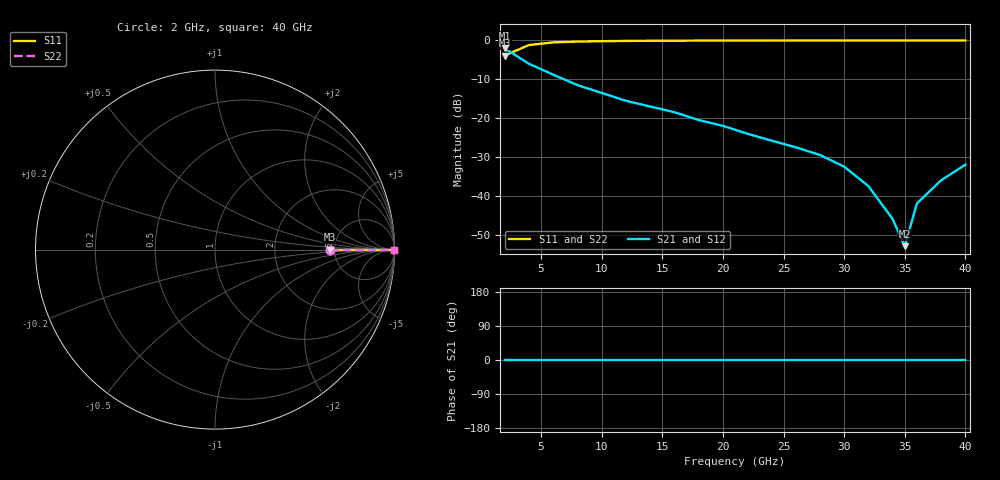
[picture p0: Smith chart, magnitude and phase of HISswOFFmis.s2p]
# GHZ S MA R 50
!Output file by Shape3_28
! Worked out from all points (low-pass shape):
!   21 points, 2 GHz to 40 GHz, reference 50 ohm
!   highest |S21| = -2.04 dB at 2 GHz (marker M1); lowest = -53.0 dB at 35 GHz (marker M2)
!   |S21| within 3 dB of the highest: start of sweep to 3.513 GHz
!   lowest |S11| = -3.9 dB at 2 GHz (marker M3), VSWR 4.52, Z = 226 + j0 ohm
!   |S11| at or under -10 dB: nowhere
!   |S22| runs from -3.9 to 0.0 dB; largest |S21 - S12| = 0
2  0.638 0.0  0.791 0.0  0.791 0.0  0.638 0.0
4  0.871 0.0  0.501 0.0  0.501 0.0  0.871 0.0
6  0.944 0.0  0.363 0.0  0.363 0.0  0.944 0.0
8  0.966 0.0  0.266 0.0  0.266 0.0  0.966 0.0
10  0.977 0.0  0.211 0.0  0.211 0.0  0.977 0.0
12  0.985 0.0  0.167 0.0  0.167 0.0  0.985 0.0
14  0.99 0.0  0.141 0.0  0.141 0.0  0.99 0.0
16  0.992 0.0  0.119 0.0  0.119 0.0  0.992 0.0
18  0.994 0.0  0.0944 0.0  0.0944 0.0  0.994 0.0
20  0.996 0.0  0.0794 0.0  0.0794 0.0  0.996 0.0
22  0.997 0.0  0.063 0.0  0.063 0.0  0.997 0.0
24  0.9975 0.0  0.0513 0.0  0.0513 0.0  0.9975 0.0
26  0.998 0.0  0.0421 0.0  0.0421 0.0  0.998 0.0
28  0.9985 0.0  0.0335 0.0  0.0335 0.0  0.9985 0.0
30  0.9986 0.0  0.0237 0.0  0.0237 0.0  0.9986 0.0
32  0.9988 0.0  0.0133 0.0  0.0133 0.0  0.9988 0.0
34  0.9989 0.0  0.005012 0.0  0.005012 0.0  0.9989 0.0
35  0.999 0.0  0.002239 0.0  0.002239 0.0  0.999 0.0
36  0.9989 0.0  0.007943 0.0  0.007943 0.0  0.9989 0.0
38  0.9988 0.0  0.0158 0.0  0.0158 0.0  0.9988 0.0
40  0.9986 0.0  0.0251 0.0  0.0251 0.0  0.9986 0.0
